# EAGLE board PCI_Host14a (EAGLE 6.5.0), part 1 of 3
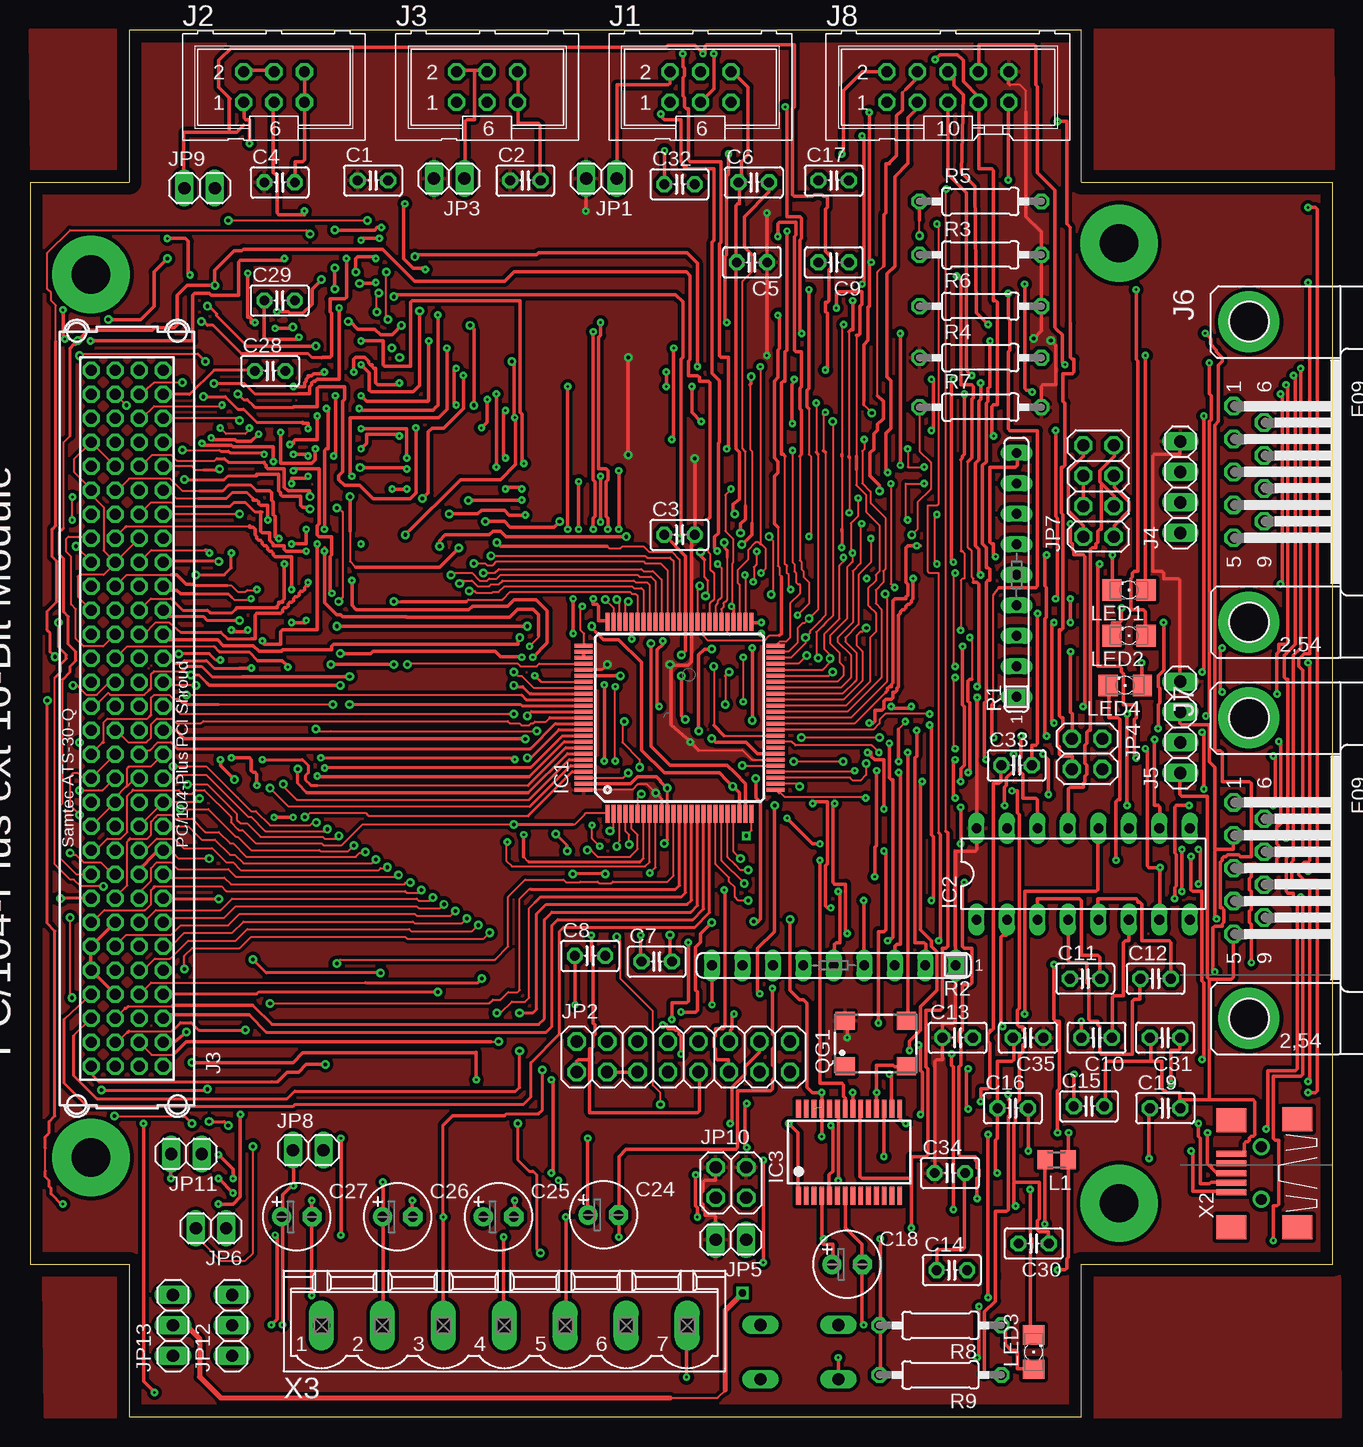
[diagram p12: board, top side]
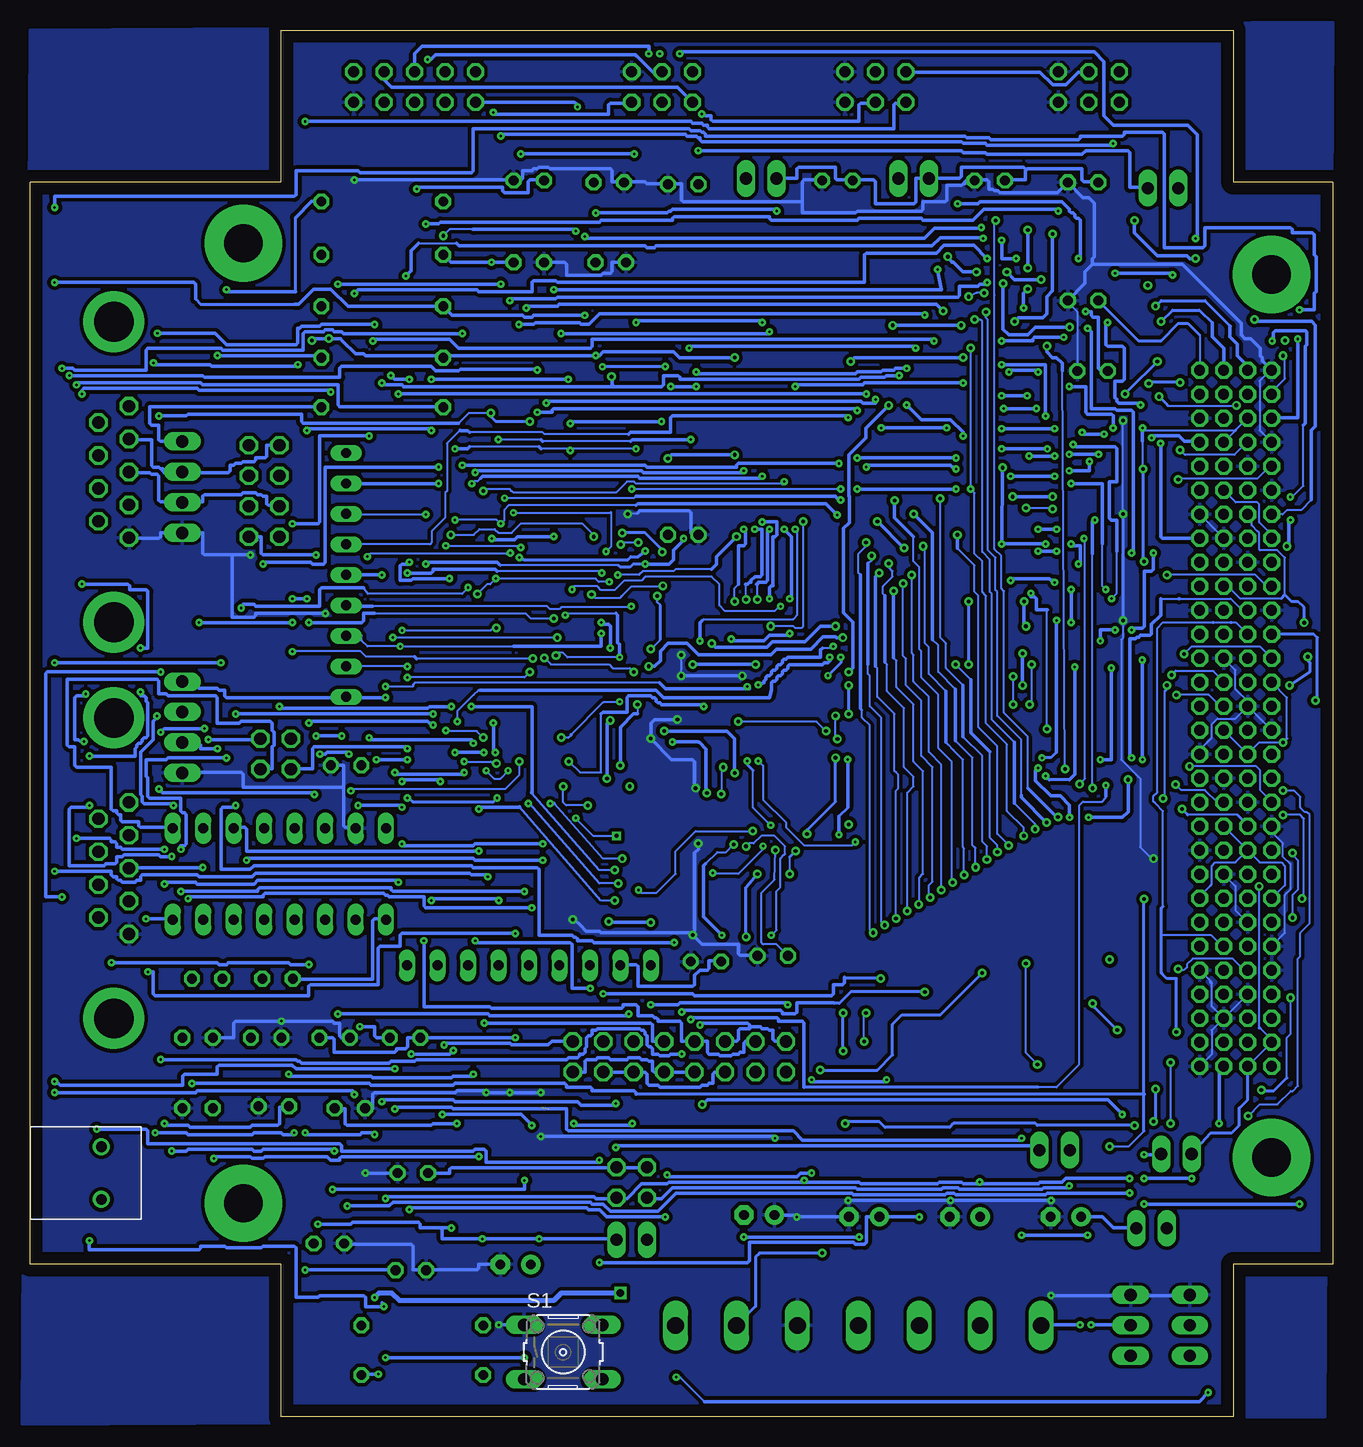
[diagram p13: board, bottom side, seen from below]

Size 108.6 x 115.57 mm. Coordinates in mm from the lower left corner, seen from the top.
Copper layers (1*16): Top 0.035mm / dielectric 1.5mm / Bottom 0.035mm
Design rules "default *": minimum track width 6mil, minimum drill 8mil, track to track 6mil, track to pad 6mil, pad to pad 8mil, via to via 8mil, smd to smd 8mil, copper to edge 40mil, drill to drill 8mil, minimum pad ring 10mil, minimum via ring 8mil, stop-mask expansion 4mil, vias tented up to drill 0mil, thermal gap 10mil
Net classes: 0 default: width 0.152 mm

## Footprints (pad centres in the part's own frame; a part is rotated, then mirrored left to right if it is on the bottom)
C025-025X050 = drill 0.813 octagon: 1 -1.27,0; 2 1.27,0
E2,5-6 = drill 0.813 pad 1.6: + -1.27,0 | drill 0.813 pad 1.6 octagon: - 1.27,0
TQFP100 = smd 1.5 x 0.35: 1 -8,6; 2 -8,5.5; 3 -8,5; 4 -8,4.5; 5 -8,4; 6 -8,3.5; 7 -8,3; 8 -8,2.5; 9 -8,2; 10 -8,1.5; 11 -8,1; 12 -8,0.5; 13 -8,0; 14 -8,-0.5; 15 -8,-1; 16 -8,-1.5; 17 -8,-2; 18 -8,-2.5; 19 -8,-3; 20 -8,-3.5; 21 -8,-4; 22 -8,-4.5; 23 -8,-5; 24 -8,-5.5; 25 -8,-6; 51 8,-6; 52 8,-5.5; 53 8,-5; 54 8,-4.5; 55 8,-4; 56 8,-3.5; 57 8,-3; 58 8,-2.5; 59 8,-2; 60 8,-1.5; 61 8,-1; 62 8,-0.5; 63 8,0; 64 8,0.5; 65 8,1; 66 8,1.5; 67 8,2; 68 8,2.5; 69 8,3; 70 8,3.5; 71 8,4; 72 8,4.5; 73 8,5; 74 8,5.5; 75 8,6 | smd 0.35 x 1.5: 26 -6,-8; 27 -5.5,-8; 28 -5,-8; 29 -4.5,-8; 30 -4,-8; 31 -3.5,-8; 32 -3,-8; 33 -2.5,-8; 34 -2,-8; 35 -1.5,-8; 36 -1,-8; 37 -0.5,-8; 38 0,-8; 39 0.5,-8; 40 1,-8; 41 1.5,-8; 42 2,-8; 43 2.5,-8; 44 3,-8; 45 3.5,-8; 46 4,-8; 47 4.5,-8; 48 5,-8; 49 5.5,-8; 50 6,-8; 76 6,8; 77 5.5,8; 78 5,8; 79 4.5,8; 80 4,8; 81 3.5,8; 82 3,8; 83 2.5,8; 84 2,8; 85 1.5,8; 86 1,8; 87 0.5,8; 88 0,8; 89 -0.5,8; 90 -1,8; 91 -1.5,8; 92 -2,8; 93 -2.5,8; 94 -3,8; 95 -3.5,8; 96 -4,8; 97 -4.5,8; 98 -5,8; 99 -5.5,8; 100 -6,8
DIL16 = drill 0.813 long: 1 -8.89,-3.81; 2 -6.35,-3.81; 3 -3.81,-3.81; 4 -1.27,-3.81; 5 1.27,-3.81; 6 3.81,-3.81; 7 6.35,-3.81; 8 8.89,-3.81; 9 8.89,3.81; 10 6.35,3.81; 11 3.81,3.81; 12 1.27,3.81; 13 -1.27,3.81; 14 -3.81,3.81; 15 -6.35,3.81; 16 -8.89,3.81
SSOP28 = smd 0.4 x 1.5: 1 -4.225,-3.625; 2 -3.575,-3.625; 3 -2.925,-3.625; 4 -2.275,-3.625; 5 -1.625,-3.625; 6 -0.975,-3.625; 7 -0.325,-3.625; 8 0.325,-3.625; 9 0.975,-3.625; 10 1.625,-3.625; 11 2.275,-3.625; 12 2.925,-3.625; 13 3.575,-3.625; 14 4.225,-3.625; 15 4.225,3.625; 16 3.575,3.625; 17 2.925,3.625; 18 2.275,3.625; 19 1.625,3.625; 20 0.975,3.625; 21 0.325,3.625; 22 -0.325,3.625; 23 -0.975,3.625; 24 -1.625,3.625; 25 -2.275,3.625; 26 -2.925,3.625; 27 -3.575,3.625; 28 -4.225,3.625
ML6 = drill 0.914 octagon: 1 -2.54,-1.27; 2 -2.54,1.27; 3 0,-1.27; 4 0,1.27; 5 2.54,-1.27; 6 2.54,1.27
1X04 = drill 1.016 long: 1 -3.81,0; 2 -1.27,0; 3 1.27,0; 4 3.81,0
F09HP = drill 1.016 octagon: 1 -5.486,-1.27; 2 -2.743,-1.27; 3 0,-1.27; 4 2.743,-1.27; 5 5.486,-1.27; 6 -4.115,1.27; 7 -1.372,1.27; 8 1.372,1.27; 9 4.115,1.27 | drill 3.302 pad 5.08: G1 -12.522,0; G2 12.522,0
ML10 = drill 0.914 octagon: 1 -5.08,-1.27; 2 -5.08,1.27; 3 -2.54,-1.27; 4 -2.54,1.27; 5 0,-1.27; 6 0,1.27; 7 2.54,-1.27; 8 2.54,1.27; 9 5.08,-1.27; 10 5.08,1.27
1X02 = drill 1.016 long: 1 -1.27,0; 2 1.27,0
2X08 = drill 1.016 octagon: 1 -8.89,-1.27; 2 -8.89,1.27; 3 -6.35,-1.27; 4 -6.35,1.27; 5 -3.81,-1.27; 6 -3.81,1.27; 7 -1.27,-1.27; 8 -1.27,1.27; 9 1.27,-1.27; 10 1.27,1.27; 11 3.81,-1.27; 12 3.81,1.27; 13 6.35,-1.27; 14 6.35,1.27; 15 8.89,-1.27; 16 8.89,1.27
2X02 = drill 1.016 octagon: 1 -1.27,-1.27; 2 -1.27,1.27; 3 1.27,-1.27; 4 1.27,1.27
2X04 = drill 1.016 octagon: 1 -3.81,-1.27; 2 -3.81,1.27; 3 -1.27,-1.27; 4 -1.27,1.27; 5 1.27,-1.27; 6 1.27,1.27; 7 3.81,-1.27; 8 3.81,1.27
1X03 = drill 1.016 long: 1 -2.54,0; 2 0,0; 3 2.54,0
M0805 = smd 1.3 x 1.6: 1 -0.95,0; 2 0.95,0
1206 = smd 1.6 x 1.803: A -1.422,0; C 1.422,0
SM77H = smd 1.6 x 1.5: 1 -2.55,-1.9; 2 2.55,-1.9; 3 2.55,1.9; 4 -2.55,1.9
SIL9 = drill 0.813 long: 1 -10.16,0; 2 -7.62,0; 3 -5.08,0; 4 -2.54,0; 5 0,0; 6 2.54,0; 7 5.08,0; 8 7.62,0; 9 10.16,0
0207/10 = drill 0.813 octagon: 1 -5.08,0; 2 5.08,0
B3F-10XX = drill 1.016 long: 1 -3.251,2.261; 2 3.251,2.261; 3 -3.251,-2.261; 4 3.251,-2.261
PC104-PLUS = drill 0.9 octagon: J3-A1 11.08,16.51; J3-A2 11.08,18.51; J3-A3 11.08,20.51; J3-A4 11.08,22.51; J3-A5 11.08,24.51; J3-A6 11.08,26.51; J3-A7 11.08,28.51; J3-A8 11.08,30.51; J3-A9 11.08,32.51; J3-A10 11.08,34.51; J3-A11 11.08,36.51; J3-A12 11.08,38.51; J3-A13 11.08,40.51; J3-A14 11.08,42.51; J3-A15 11.08,44.51; J3-A16 11.08,46.51; J3-A17 11.08,48.51; J3-A18 11.08,50.51; J3-A19 11.08,52.51; J3-A20 11.08,54.51; J3-A21 11.08,56.51; J3-A22 11.08,58.51; J3-A23 11.08,60.51; J3-A24 11.08,62.51; J3-A25 11.08,64.51; J3-A26 11.08,66.51; J3-A27 11.08,68.51; J3-A28 11.08,70.51; J3-A29 11.08,72.51; J3-A30 11.08,74.51; J3-B1 9.08,16.51; J3-B2 9.08,18.51; J3-B3 9.08,20.51; J3-B4 9.08,22.51; J3-B5 9.08,24.51; J3-B6 9.08,26.51; J3-B7 9.08,28.51; J3-B8 9.08,30.51; J3-B9 9.08,32.51; J3-B10 9.08,34.51; J3-B11 9.08,36.51; J3-B12 9.08,38.51; J3-B13 9.08,40.51; J3-B14 9.08,42.51; J3-B15 9.08,44.51; J3-B16 9.08,46.51; J3-B17 9.08,48.51; J3-B18 9.08,50.51; J3-B19 9.08,52.51; J3-B20 9.08,54.51; J3-B21 9.08,56.51; J3-B22 9.08,58.51; J3-B23 9.08,60.51; J3-B24 9.08,62.51; J3-B25 9.08,64.51; J3-B26 9.08,66.51; J3-B27 9.08,68.51; J3-B28 9.08,70.51; J3-B29 9.08,72.51; J3-B30 9.08,74.51; J3-C1 7.08,16.51; J3-C2 7.08,18.51; J3-C3 7.08,20.51; J3-C4 7.08,22.51; J3-C5 7.08,24.51; J3-C6 7.08,26.51; J3-C7 7.08,28.51; J3-C8 7.08,30.51; J3-C9 7.08,32.51; J3-C10 7.08,34.51; J3-C11 7.08,36.51; J3-C12 7.08,38.51; J3-C13 7.08,40.51; J3-C14 7.08,42.51; J3-C15 7.08,44.51; J3-C16 7.08,46.51; J3-C17 7.08,48.51; J3-C18 7.08,50.51; J3-C19 7.08,52.51; J3-C20 7.08,54.51; J3-C21 7.08,56.51; J3-C22 7.08,58.51; J3-C23 7.08,60.51; J3-C24 7.08,62.51; J3-C25 7.08,64.51; J3-C26 7.08,66.51; J3-C27 7.08,68.51; J3-C28 7.08,70.51; J3-C29 7.08,72.51; J3-C30 7.08,74.51; J3-D1 5.08,16.51; J3-D2 5.08,18.51; J3-D3 5.08,20.51; J3-D4 5.08,22.51; J3-D5 5.08,24.51; J3-D6 5.08,26.51; J3-D7 5.08,28.51; J3-D8 5.08,30.51; J3-D9 5.08,32.51; J3-D10 5.08,34.51; J3-D11 5.08,36.51; J3-D12 5.08,38.51; J3-D13 5.08,40.51; J3-D14 5.08,42.51; J3-D15 5.08,44.51; J3-D16 5.08,46.51; J3-D17 5.08,48.51; J3-D18 5.08,50.51; J3-D19 5.08,52.51; J3-D20 5.08,54.51; J3-D21 5.08,56.51; J3-D22 5.08,58.51; J3-D23 5.08,60.51; J3-D24 5.08,62.51; J3-D25 5.08,64.51; J3-D26 5.08,66.51; J3-D27 5.08,68.51; J3-D28 5.08,70.51; J3-D29 5.08,72.51; J3-D30 5.08,74.51 | drill 3.2 pad 6.452: P$1 5.085,82.5; P$2 5.085,8.9; P$3 90.785,5.1; P$4 90.785,85.1
USB-MB-S = smd 2.5 x 0.5: D+ 2.5,0; D- 2.5,0.8; GND 2.5,-1.6; ID 2.5,-0.8; VBUS 2.5,1.6 | smd 2.5 x 2: P$1 -3,-4.5; P$2 -3,4.5; P$3 2.5,-4.4; P$4 2.5,4.5 | drill 0.9: P$5 0,2.2; P$6 0,-2.2
MSTBV7 = drill 1.397 long: 1 -15.24,0; 2 -10.16,0; 3 -5.08,0; 4 0,0; 5 5.08,0; 6 10.16,0; 7 15.24,0

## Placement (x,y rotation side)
C1  100nF  [C025-025X050]  28.59,103.03 0 top
C2  100nF  [C025-025X050]  41.29,103.03 0 top
C3  100nF  [C025-025X050]  54.15,73.5 0 top
C4  100nF  [C025-025X050]  20.81,102.87 0 top
C5  100nF  [C025-025X050]  60.18,96.2 180 top
C6  100nF  [C025-025X050]  60.34,102.87 0 top
C7  10n  [C025-025X050]  52.24,37.94 0 top
C8  10n  [C025-025X050]  46.69,38.42 0 top
C9  10n  [C025-025X050]  67.01,96.2 180 top
C10  1u  [C025-025X050]  88.92,31.59 180 top
C11  1u  [C025-025X050]  87.96,36.51 0 top
C12  1u  [C025-025X050]  93.84,36.51 0 top
C13  1u  [C025-025X050]  77.33,31.59 0 top
C14  10n  [C025-025X050]  76.85,12.22 0 top
C15  47p  [C025-025X050]  88.28,25.88 0 top
C16  47p  [C025-025X050]  81.93,25.72 0 top
C17  100n  [C025-025X050]  67.01,103.03 0 top
C18  4.7u  [E2,5-6]  68.12,12.7 0 top
C19  100n  [C025-025X050]  94.63,25.72 0 top
C24  47u  [E2,5-6]  47.8,16.83 0 top
C25  47u  [E2,5-6]  39.07,16.67 0 top
C26  47u  [E2,5-6]  30.65,16.67 0 top
C27  47u  [E2,5-6]  22.24,16.67 0 top
C28  100n  [C025-025X050]  20.02,87.15 0 top
C29  100n  [C025-025X050]  20.81,93.03 0 top
C30  100n  [C025-025X050]  83.68,14.45 180 top
C31  100n  [C025-025X050]  94.63,31.59 180 top
C32  100n  [C025-025X050]  54.15,102.71 0 top
C33  100n  [C025-025X050]  82.25,54.29 0 top
C34  100n  [C025-025X050]  76.69,20.32 0 top
C35  100n  [C025-025X050]  83.2,31.59 180 top
IC1  ATMEGA640-16AI  [TQFP100]  54.15,58.26 90 top
IC2  MAX232  [DIL16]  87.8,45.24 0 top
IC3  FT232RL  [SSOP28]  68.28,22.07 0 top
J1  [ML6]  55.9,110.81 0 top
J2  [ML6]  20.34,110.81 0 top
J3  [ML6]  38.12,110.81 0 top
J4  [1X04]  95.9,77.47 90 top
J5  [1X04]  95.9,57.47 90 top
J6  [F09HP]  101.61,78.74 270 top
J7  [F09HP]  101.61,45.72 270 top
J8  [ML10]  76.53,110.81 0 top
JP1  [1X02]  47.64,103.19 180 top
JP2  [2X08]  54.47,30 0 top
JP3  [1X02]  34.94,103.19 180 top
JP4  [2X02]  88.12,55.24 270 top
JP5  [1X02]  58.44,14.76 180 top
JP6  [1X02]  15.1,15.72 180 top
JP7  [2X04]  89.07,77.15 90 top
JP8  [1X02]  23.19,22.23 0 top
JP9  [1X02]  14.14,102.39 0 top
JP10  [2X02]  58.43,19.53 0 top
JP11  [1X02]  13.03,21.91 180 top
JP12  [1X03]  16.84,7.62 90 top
JP13  [1X03]  11.92,7.62 90 top
L1  [M0805]  85.58,21.43 180 top
LED1  gr  [1206]  91.61,68.9 180 top
LED2  [1206]  91.61,65.09 180 top
LED3  rt  [1206]  83.68,5.4 90 top
LED4  or  [1206]  91.3,60.96 180 top
QG1  SM77H  [SM77H]  70.5,31.11 0 top
R1  4K7  [SIL9]  82.25,70.17 90 top
R2  4k7  [SIL9]  67.01,37.62 180 top
R3  10k  [0207/10]  79.23,96.84 0 top
R4  220R  [0207/10]  79.23,88.27 0 top
R5  220R  [0207/10]  79.23,101.28 0 top
R6  10k  [0207/10]  79.23,92.55 0 top
R7  10k  [0207/10]  79.23,84.14 0 top
R8  220R  [0207/10]  75.9,7.62 180 top
R9  220R  [0207/10]  75.9,3.49 180 top
S1  [B3F-10XX]  64.15,5.4 0 bottom
X1  PC104_PLUS_USB_SUBD  [PC104-PLUS]  0.01,12.7 0 top
X2  USB-MB-S  [USB-MB-S]  102.65,20.32 180 top
X3  MSTBV7  [MSTBV7]  39.54,7.62 0 top

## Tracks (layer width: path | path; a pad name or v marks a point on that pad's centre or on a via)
AD00  (via drill 0.3)
  Top 0.152: v25.57,37.78 25.89,38.1 38.75,38.1 39.86,39.21 39.86,43.34 41.29,44.77 44.47,44.77 44.7,44.53 45.81,44.53 45.89,44.61 47.32,44.61 47.48,44.45 48.43,44.45 48.59,44.61 53.15,44.61 53.65,45.11 IC1.12
  Top 0.254: X1.J3-D1 5.09,28.57 5.73,27.94 20.18,27.94 20.65,27.94
  Top 0.305: v24.62,29.37 23.03,29.37 22.4,28.73 21.45,28.73 20.65,27.94
  Bottom 0.152: v24.62,29.37 25.57,30.32 v25.57,37.78
AD01  (via drill 0.3)
  Top 0.152: 7.25,31.21 8.11,32.07 | 8.27,32.15 11.84,32.15 | v20.02,34.45 38.27,34.45 38.59,34.77 39.23,34.77 39.86,35.4 40.66,35.4 40.81,35.56 40.81,43.18 41.61,43.97 41.77,43.97
  Top 0.254: X1.J3-C2 7.25,31.21 | 8.11,32.07 8.19,32.07 8.27,32.15 | 11.84,32.15 12.56,32.86 13.43,32.86 14.06,32.23 v17.95,32.23 | IC1.13 54.15,44.29 53.83,43.97 41.77,43.97
  Top 0.305: v20.02,34.45 | v20.02,34.45 19.98,34.49
  Bottom 0.254: v17.95,32.23 19.86,34.13
  Bottom 0.305: 19.86,34.13 20.02,34.29 v20.02,34.45
AD02  (via drill 0.3)
  Top 0.152: 11.92,30.16 10.14,30.16 X1.J3-B2 | 42.08,42.86 41.61,42.39 41.61,34.92 41.29,34.61 40.18,34.61 39.23,33.66 v38.91,33.66 | 38.43,31.27 v39.07,31.27
  Top 0.254: IC1.14 54.65,43.68 54.31,43.34 42.56,43.34 42.08,42.86
  Top 0.305: 38.43,31.27 13.03,31.27 11.92,30.16
  Bottom 0.152: v38.91,33.66 39.07,33.5 v39.07,31.27
AD03  (via drill 0.3)
  Top 0.152: 3.67,31.78 X1.J3-D3
  Top 0.254: IC1.15 55.15,43.07 54.78,42.7 43.04,42.7 | 3.67,31.78 3.67,28.42 5.57,26.51 21.45,26.51 22.08,27.15 40.5,27.15 40.81,27.46 v40.81,30.48 | v40.81,33.66 41.92,33.66 42.24,33.97 42.24,41.91 43.04,42.7 | 43.04,42.7
  Bottom 0.254: v40.81,30.48 v40.81,33.66
AD04
  Top 0.152: 8.19,34.21 11.84,34.21 | X1.J3-C3 7.94,34.05
  Top 0.254: IC1.16 55.65,42.62 55.1,42.07 43.51,42.07 42.88,41.43 42.88,33.18 42.4,32.7 20.17,32.7 18.58,34.29 | 8.19,34.21 8.03,34.05 7.94,34.05
  Top 0.305: 18.58,34.29 11.92,34.29 11.84,34.21
AD05
  Top 0.254: IC1.17 56.15,42.32 55.26,41.43 43.99,41.43 43.51,40.96 43.51,32.54 43.04,32.07 19.7,32.07 18.27,33.5
  Top 0.305: 18.27,33.5 11.38,33.5 X1.J3-A3
AD06
  Top 0.152: 2.87,33.15 X1.J3-D4
  Top 0.254: IC1.18 56.65,42.03 55.42,40.8 44.47,40.8 44.15,40.48 44.15,31.91 41.77,29.53 41.77,26.67 41.13,26.04 22.08,26.04 21.92,25.88 4.78,25.88 2.87,27.78 2.87,33.15
AD07  (via drill 0.2, 0.3)
  Top 0.152: 9.11,35.21 10.1,36.2 27.96,36.2 | IC1.27 63.91,52.76 v64.15,52.53
  Top 0.254: X1.J3-B4 9.11,35.21 | 27.96,36.2 37.34,36.2 v37.68,36.54
  Top 0.305: v62.09,50.96 62.04,50.95 62.04,40.44 60.66,39.05 60.66,35.42 v60.82,35.25
  Bottom 0.152: v64.15,52.53 64.15,51.2 63.91,50.96 v62.09,50.96
  Bottom 0.254: v37.68,36.54 40.62,36.54 40.71,36.63
  Bottom 0.305: v60.82,35.25 53.36,35.25 53.2,35.1 41.77,35.1 41.62,35.25 41.62,36.02 40.86,36.02 40.71,36.17 40.71,36.63
AD08  (via drill 0.3)
  Top 0.152: 51.13,72.55 51.61,72.07 53.51,72.07 54.15,71.44 IC1.63 | IC1.63 | 51.13,72.55 | v12.87,37.31 12.87,38.42 13.51,39.05 17.48,39.05 18.43,40 31.29,40 31.45,39.85 37.82,39.85 v38.31,40.34 | 48.12,72.55 48.27,72.39 | 48.27,72.39 | 48.27,72.39 49.23,72.39 49.39,72.55 51.13,72.55
  Top 0.305: v38.91,72.87 39.23,72.55 48.12,72.55
  Bottom 0.152: 7.38,37.21 8.35,38.18 11.68,38.18 12.16,37.7 12.16,37.47 12.4,37.23 12.64,37.23 | v38.31,40.34 38.59,40.62 38.59,57.63 39.23,58.26 39.23,58.9 39.38,59.05 | 39.38,70.17 39.54,70.33 39.54,71.91 38.91,72.55 v38.91,72.87
  Bottom 0.254: X1.J3-C5 7.38,37.21 | 12.64,37.23 12.71,37.31 v12.87,37.31
  Bottom 0.305: 39.38,59.05 39.38,70.17
AD09  (via drill 0.3)
  Top 0.152: X1.J3-B5 9.44,37.21 10.41,38.18 11.68,38.18 13.19,39.69 17.16,39.69 18.11,40.64 31.61,40.64 31.77,40.48 36.87,40.48 v37.36,40.97 | v38.43,71.75 51.29,71.75 51.45,71.6 53.36,71.6 53.67,71.28 53.65,71.25 IC1.64
  Bottom 0.152: v37.36,40.97 37.64,41.25 37.64,58.26 38.59,59.21 38.59,61.75 38.75,61.91 38.75,62.55 38.75,62.71 | 38.75,71.12 38.43,71.44 v38.43,71.75
  Bottom 0.305: 38.75,62.71 38.75,71.12
AD10  (via drill 0.3)
  Top 0.152: 7.09,39.23 8.03,40.16 11.76,40.16 12.08,40.48 | v37,71.12 37.32,71.12 | 37.32,71.12 | 37.32,71.12 37.96,71.12 38.12,70.96 38.59,70.96 38.91,71.28 51.13,71.28 51.29,71.12 52.56,71.12 53.15,70.53 IC1.65 | 12.08,40.48 | 12.08,40.48 12.56,40.96 16.53,40.96 17.48,41.91 32.08,41.91 32.24,41.75 35.06,41.75 v35.46,42.15
  Top 0.254: X1.J3-C6 7.09,39.23
  Bottom 0.152: 37.32,68.42 37.48,68.58 37.48,69.22 36.69,70.01 36.69,70.48 37,70.8 v37,71.12 | 37.32,62.86 37.16,62.71 37.16,60.48 35.73,59.05 35.73,54.13 34.94,53.34 34.94,52.55 35.46,52.02 v35.46,42.15
  Bottom 0.305: 37.32,62.86 37.32,68.42
AD11  (via drill 0.3)
  Top 0.152: 52.24,70.17 | v37.8,70.33 38.75,70.33 39.07,70.64 50.97,70.64 51.13,70.48 51.93,70.48 52.24,70.17 | X1.J3-A6 11.76,39.21 12.87,40.32 16.84,40.32 17.8,41.27 31.92,41.27 32.08,41.12 36.01,41.12 v36.41,41.52 | IC1.66 52.65,69.76 52.24,70.17
  Bottom 0.152: v37.8,70.33 | 38.12,70.01 v37.8,70.33 | 38.12,62.55 37.96,62.39 37.96,60.01 36.53,58.58 36.53,53.82 36.37,53.66 | 36.37,53.66 | 36.37,53.66 36.21,53.5 36.21,52.39 36.41,52.19 v36.41,41.52
  Bottom 0.305: 38.12,62.55 38.12,70.01
AD12  (via drill 0.3)
  Top 0.152: 5.19,41.21 6.21,42.23 9.54,42.23 9.62,42.23 10.1,42.7 10.1,43.89 10.33,44.13 | 10.41,44.21 15.97,44.21 16.37,43.81 31.29,43.81 31.45,43.66 32.37,43.66 v32.62,43.91 | v35.1,70.17 35.26,70.33 36.84,70.33 37.48,69.69 38.12,69.69 38.27,69.85 38.91,69.85 39.23,70.17 50.66,70.17 50.81,70.01 51.77,70.01 52.15,69.63 IC1.67
  Top 0.254: X1.J3-D7 5.19,41.21 | 10.33,44.13 | 10.33,44.13 10.41,44.21
  Bottom 0.152: v32.62,43.91 32.62,54.36 33.67,55.4 33.67,60.01 34.94,61.28 34.94,63.5 35.1,63.66 v35.1,70.17
AD13  (via drill 0.3)
  Top 0.152: X1.J3-B7 9.48,41.21 10.49,42.23 15.89,42.23 16.84,43.18 32.24,43.18 32.4,43.02 33.33,43.02 v33.57,43.27 | v35.81,69.45 36.05,69.69 36.84,69.69 37.32,69.22 38.27,69.22 38.43,69.37 39.07,69.37 39.38,69.69 50.34,69.69 50.5,69.53 51.45,69.53 51.65,69.33 IC1.68
  Bottom 0.152: v35.81,69.45 35.81,63.42 35.58,63.18 35.58,60.96 34.3,59.69 34.3,55.09 33.35,54.13 33.35,44.61 33.67,44.29 33.67,43.36 v33.57,43.27
AD14  (via drill 0.3)
  Top 0.152: 38.59,68.74 39.07,68.74 39.54,69.22 50.18,69.22 50.34,69.06 50.97,69.06 51.15,68.88 IC1.69 | 38.59,68.74 | 38.59,68.74 38.51,68.66 37.24,68.66 37.08,68.82 v36.61,68.82 | X1.J3-A7 11.54,41.21 11.92,41.59 16.21,41.59 17.16,42.55 32.24,42.55 32.4,42.39 34.19,42.39 v34.52,42.71
  Bottom 0.152: v34.52,42.71 34.46,42.76 34.46,44.93 34.15,45.24 34.15,53.82 34.94,54.61 34.94,59.37 36.37,60.8 36.37,63.02 36.61,63.26
  Bottom 0.305: 36.61,63.26 v36.61,68.82
AD15  (via drill 0.3)
  Top 0.152: 7.09,43.35 8.11,44.29 8.11,47.94 8.27,48.1 | 8.35,48.18 9.78,48.18 10.1,48.5 10.1,49.61 10.49,50.01 10.65,50.17 11.76,50.17 12.08,49.85 13.51,49.85 14.62,48.74 15.73,48.74 16.68,47.78 16.92,47.78 18.03,46.67 27.16,46.67 27.48,46.99 27.88,46.99 v27.96,47.07 | IC1.79 42.46,62.76 42.24,62.55 40.89,62.55 40.66,62.79 31.53,62.79 v31.45,62.71
  Top 0.254: X1.J3-C8 7.09,43.35 | 8.27,48.1 | 8.27,48.1 8.35,48.18
  Bottom 0.152: v27.96,47.07 27.96,47.62 28.59,48.26 28.59,55.4 | 30.18,61.44 v31.45,62.71
  Bottom 0.305: 28.59,55.4 30.18,56.99 30.18,61.44
AD16
  Top 0.152: 9.45,55.56 10.02,55.56 10.65,56.2 11.76,56.2
  Top 0.254: X1.J3-B14 9.45,55.56 | 11.76,56.2 12.28,55.68 41.72,55.68 43.82,57.78 43.85,57.76 IC1.89
AD17
  Top 0.152: 7.18,57.21 8.19,56.2 9.7,56.2 10.1,56.59 10.1,57.71 10.57,58.18 11.84,58.18 12.24,57.78 14.24,57.78 14.44,57.98 39.82,57.98 40.02,57.78 40.81,57.78 40.97,57.63 41.61,57.63 41.77,57.78 41.92,57.78 42.08,57.94 43.04,57.94 43.35,58.26
  Top 0.254: X1.J3-C15 7.18,57.21 | IC1.88 43.35,58.26
AD18  (via drill 0.3)
  Top 0.254: X1.J3-A15 12.18,57.21 | 41.77,58.74 v41.45,58.42 41.79,58.76 IC1.87
  Top 0.305: 12.18,57.21 12.87,56.52 41.27,56.52 v41.29,56.5
  Bottom 0.152: v41.45,58.42 41.45,56.65 v41.29,56.5
AD19  (via drill 0.3)
  Top 0.152: X1.J3-D16 5.41,59.21 6.52,60.33 6.68,60.17 9.54,60.17 9.94,60.56 | 10.1,60.72 10.1,61.91 10.33,62.15 12.71,62.15 | v26.64,61.69 26.39,61.69 26.37,61.67
  Top 0.254: 9.94,60.56 | 9.94,60.56 10.1,60.72 | 12.71,62.15 13.11,62.55 14.3,62.55 15.18,61.67 17.72,61.67 | v26.64,59.37 40.89,59.37 41,59.26 IC1.86 | 26.45,61.67
  Top 0.305: 17.72,61.67 26.37,61.67 26.45,61.67
  Bottom 0.152: v26.64,61.69 v26.64,59.37
AD20  (via drill 0.3)
  Top 0.152: v13.03,60.17 40.97,60.17
  Top 0.254: 40.97,60.17 41.37,59.77 IC1.85
  Bottom 0.152: 9.38,59.21 10.33,60.17 v13.03,60.17
  Bottom 0.254: X1.J3-B16 9.38,59.21
AD21  (via drill 0.3)
  Top 0.152: v40.34,58.58 12.52,58.58 11.89,59.21 X1.J3-A16
  Top 0.254: 41.79,60.26 IC1.84 | 41.79,60.26 41.79,60.27 | 41.33,60.58 | 41.33,60.58 41.07,60.84 40.46,60.84 v40.34,60.96 | 41.79,60.26 41.65,60.26 41.33,60.58
  Bottom 0.254: v40.34,58.58 v40.34,60.96
AD22  (via drill 0.3)
  Top 0.152: X1.J3-C17 6.61,61.21 5.57,60.17 4.7,60.17 3.9,60.96 | IC1.83 41.97,60.76 40.97,61.75 40.66,61.75 v40.34,62.07 | 2.16,89.61 2.16,92.63 1.76,93.03 1.76,93.66 1.44,93.98 1.44,97 3.35,98.9 23.03,98.9 v23.35,98.58
  Top 0.254: 2.16,89.61 2.16,74.3 1.84,73.98 1.84,71.68 2.24,71.28 2.24,67.94 1.44,67.15 1.44,65.56 1.68,65.33 1.68,63.74 v2.08,63.34 | v3.59,60.96 3.9,60.96
  Top 0.305: v37,84.3 37,90.65 v36.69,90.96 | v26.53,91.28 26.69,91.28 27.32,90.65 28.75,90.65 29.23,90.17 30.18,90.17 v30.97,90.96
  Bottom 0.254: v3.59,60.96 1.92,62.07 1.92,62.86 2.08,63.02 v2.08,63.34
  Bottom 0.305: v37,84.3 38.91,82.39 38.91,81.6 40.34,80.17 40.34,76.74 40.3,76.7 40.3,74.51 40.77,74.04 40.77,67.01 39.98,66.22 39.98,62.43 v40.34,62.07 | v30.97,90.96 v36.69,90.96 | v23.35,98.58 23.35,93.82 23.83,93.34 23.83,91.92 24.14,91.6 26.21,91.6 v26.53,91.28
AD23  (via drill 0.2, 0.3)
  Top 0.152: 42.59,61.26 IC1.82
  Top 0.254: v13.43,61.83 14.07,61.83 14.78,61.12 | v42.08,61.76 42.08,61.77 42.59,61.26
  Top 0.305: v25.86,60.96 25.54,60.96 14.94,60.96 14.78,61.12 | v25.86,63.61 28.38,63.61 28.59,63.82 38.75,63.82 39.23,63.34 40.97,63.34 v41.01,63.3
  Bottom 0.152: 9.1,61.31 9.94,62.15 13.11,62.15
  Bottom 0.254: X1.J3-B17 9.1,61.31 | 13.11,62.15 v13.43,61.83 | v41.01,63.3 41.01,62.83 v42.08,61.76
  Bottom 0.305: v25.86,60.96 v25.86,63.61
AD24  (via drill 0.3)
  Top 0.152: v57.01,62.55 57.01,57.63 | 57.87,56.76 IC1.35
  Top 0.305: X1.J3-A19 11.16,65.21 11.6,64.77 15.65,64.77 16.12,64.27 18.61,64.27 19.09,63.82 20.97,63.82 21.05,63.91 25.16,63.91 25.16,64.21 25.31,64.36 40.71,64.36 40.71,64.82 v40.83,64.93 | 57.01,57.63 57.87,56.76
  Bottom 0.305: v57.01,62.55 56.53,62.55 56.05,63.02 56.05,63.82 55.42,64.45 53.83,64.45 52.88,63.5 46.85,63.5 46.37,63.98 43.51,63.98 42.48,65.01 41.45,65.01 41.37,64.93 v40.83,64.93
AD25  (via drill 0.2)
  Top 0.152: IC1.36 70.29,57.26 70.82,57.78 70.82,58.1 71.29,58.58 v74.99,58.58 v75,58.57
  Top 0.305: v91.45,50.95 v91.45,58.57 | v54.88,39.52 54.88,34.65 54.73,34.49 53.51,34.49 v53.51,33.12 | v18.91,52.63 18.91,53.54 18.76,53.7 18.61,53.7 18.46,53.85 18.46,54.76 18.3,54.92 v16.78,54.92
  Bottom 0.152: 7.63,67.31 8.51,68.18 12.79,68.18 | 18.91,51.71 18.91,51.59 19.22,51.28 20.81,51.28 21.13,50.96 21.13,29.37 23.03,27.46 24.53,27.46 24.55,27.48 | 14.34,68.17 12.82,68.17
  Bottom 0.254: 7.63,67.31 7.19,67.31 X1.J3-C20 | 24.55,27.48 44.06,27.48
  Bottom 0.305: v91.45,58.57 v75,58.57 | v91.45,50.95 91.61,50.8 92.52,50.8 92.67,50.65 92.67,45.62 90.24,45.62 89.93,45.92 71.8,45.92 71.64,45.77 66.31,45.77 66.16,45.62 66.16,40.13 63.41,40.13 63.26,39.98 63.11,39.98 62.96,39.83 62.96,39.67 61.74,39.67 61.59,39.52 v54.88,39.52 | v53.51,33.12 53.36,33.27 46.34,33.27 46.19,33.12 46.19,32.97 44.21,32.97 44.06,32.82 44.06,27.48 | 18.91,51.71 v18.91,52.63 | 14.34,68.17 14.34,66.8 15.1,66.04 15.1,65.28 15.26,65.13 16.02,65.13 16.17,64.97 16.32,64.97 16.47,64.82 16.93,64.82 16.93,55.07 v16.78,54.92 | 12.82,68.17 12.79,68.18
AD26  (via drill 0.2)
  Top 0.152: X1.J3-B20 10.07,68.18 11.76,68.18 | 67.68,90.88 67.68,80.21 | 67.69,80.06 67.69,73.97 | IC1.37 68.73,57.76 71.29,60.33 | 71.29,60.33 | 71.29,60.33 71.35,60.39 71.45,60.48
  Top 0.254: 11.76,68.18 12.71,67.23 14.78,67.23 15.02,66.99 16.84,66.99 17.16,67.31 | 67.68,73.81 67.68,72.6 v67.67,72.43
  Top 0.305: v24.7,84.02 24.86,83.87 24.86,80.67 24.7,80.67 24.55,80.52 v24.55,73.97 | v67.83,91.03 67.68,90.88 | 67.68,80.21 67.69,80.06 | 67.69,73.97 67.68,73.81 | 74.23,72.59 v73.93,72.59 73.17,72.59 73.02,72.44 73.02,69.55 73.17,69.39 73.17,68.48 73.02,68.33 73.02,68.17 72.1,68.17 71.95,68.02 71.95,61.16 71.8,61.01 71.8,60.86 71.64,60.86 71.49,60.71 71.49,60.55 71.34,60.4 71.35,60.39 | v34,91.82 34,84.31 33.83,84.14 | 33.83,84.14 | 33.83,84.14 33.59,83.9 27.56,83.9 v27.44,84.02 | v21.2,71.07 21.2,68.17 21.05,68.02 21.05,67.87 20.74,67.87 20.74,67.72 20.59,67.56 20.59,67.41 17.24,67.41 17.16,67.31 | v21.81,72.75 23.03,72.75 v23.03,73.97
  Bottom 0.152: 67.96,72.55 73.89,72.55 v73.93,72.59
  Bottom 0.254: v67.67,72.43 67.85,72.43 67.96,72.55
  Bottom 0.305: v24.7,84.02 v27.44,84.02 | v67.83,91.03 66.61,91.03 66.46,91.19 62.8,91.19 62.65,91.03 62.02,91.03 61.13,91.92 34.1,91.92 v34,91.82 | v21.2,71.07 21.05,71.22 21.05,72.59 21.66,72.59 v21.81,72.75 | v23.03,73.97 v24.55,73.97
AD27  (via drill 0.2, 0.3)
  Top 0.152: IC1.38 | 68.3,79.91 v68.3,75.34 v68.29,75.34 | 68.29,90.42 68.29,80.06 | IC1.38 68.44,58.26 71.45,61.28 71.45,68.42 v71.29,68.58 | v60.58,72.1 60.58,71.04 60.34,70.8 60.34,69.62 v60.3,69.58
  Top 0.254: v13.83,70.17 16.21,70.17 16.78,70.74 v16.78,71.98
  Top 0.305: 68.29,80.06 68.3,79.91 | 68.29,90.42 68.44,90.58 68.59,90.58 v68.59,93.02 | v20.43,90.71 21.83,90.71 v21.92,90.81 | v27.48,94.46 28.74,94.46 v28.82,94.54
  Bottom 0.152: X1.J3-D21 5.49,69.21 6.44,70.17 v13.83,70.17 | 68.3,75.56 68.29,75.56 v68.29,75.34 v68.28,75.34 60.24,75.34 60.17,75.41 60.17,72.51 v60.58,72.1 | v60.3,69.58 61.19,69.58 61.29,69.69 | 61.29,69.69 | 61.29,69.69 61.45,69.85 v69.76,69.85 70.23,69.37 70.5,69.37 v71.29,68.58
  Bottom 0.305: v68.59,93.02 68.44,93.17 64.78,93.17 64.63,93.32 31.26,93.32 31.11,93.47 31.11,94.23 29.58,94.23 29.43,94.39 28.97,94.39 v28.82,94.54 | v16.78,71.98 16.63,71.98 16.63,83.72 16.78,83.87 18,83.87 18.15,84.02 20.13,84.02 20.13,90.41 v20.43,90.71 | v21.92,90.81 24.78,90.81 25.41,90.17 27,90.17 27.48,90.65 v27.48,94.46
AD28  (via drill 0.2)
  Top 0.152: X1.J3-C21 8.05,70.17 11.76,70.17 | IC1.39 68.14,58.76 68.75,59.37 70.98,61.59 70.98,67.31 70.5,67.79 70.5,68.9 71.14,69.53 71.14,70.48 71.29,70.64 71.29,74.93 70.08,76.14 | v69.55,81.43 69.55,80.64 69.39,80.49 69.39,77.79 70.08,77.09 70.08,76.14 | 16.45,69.29 16.76,69.29 17.32,68.74 17.95,68.74 18.11,68.9 18.88,68.9 v18.92,68.94 | 70.08,76.14
  Top 0.254: 13.67,69.29 16.45,69.29
  Top 0.305: v53.51,81.43 53.66,81.59 v53.66,89.05 | v26.84,78.38 26.69,78.54 26.69,83.26 34.06,83.26 34.78,83.98 | v23.18,78.38 23.03,78.23 21.81,78.23 v21.81,77.78 | 34.78,83.98 34.78,89.03 v34.76,89.05 | 34.78,83.98 | 11.76,70.17 12.24,70.17 13.03,69.37 13.59,69.37 13.67,69.29
  Bottom 0.152: 66,81.43 v69.55,81.43 | 58.54,81.28 65.85,81.28 | 19.22,72.75 19.22,69.23 v18.92,68.94
  Bottom 0.305: 65.85,81.28 66,81.43 | 58.54,81.28 58.38,81.43 v53.51,81.43 | v53.66,89.05 53.51,89.2 34.91,89.2 v34.76,89.05 | v23.18,78.38 v26.84,78.38 | 19.22,72.75 19.22,77.78 v21.81,77.78
AD29  (via drill 0.2, 0.3)
  Top 0.152: 68.9,90.12 68.9,80.06 | IC1.40 68.01,59.26 70.02,61.28 70.02,64.93 70.5,65.41 70.5,66.99 70.02,67.47 | 68.89,78.96 68.89,77.65 69.71,76.84 69.71,75.41 70.34,74.77 | 70.02,67.47 69.86,67.63 69.86,69.06 70.5,69.69 70.5,70.17 70.82,70.48 70.82,74.3 70.34,74.77 | 70.02,67.47 | 16.78,68.33 | 16.78,68.33 17,68.1 18.35,68.1 v18.43,68.18 | 70.34,74.77
  Top 0.254: X1.J3-A21 11.41,68.9 | 13.51,68.58 16.53,68.58 16.78,68.33
  Top 0.305: v23.94,83.41 23.94,81.43 22.11,81.43 21.96,81.28 21.96,81.13 21.66,81.13 v21.65,81.03 | v67.22,92.41 67.22,93.62 67.38,93.78 69.36,93.78 69.36,92.71 69.2,92.56 69.2,90.27 69.05,90.12 68.9,90.12 | 68.9,80.06 68.89,78.96 | v27.6,87.68 28.27,87.01 28.27,85.57 28.43,85.41 31.92,85.41 32.48,85.96 v32.48,92.15 | 11.41,68.9 12.24,68.9 12.56,68.58 13.51,68.58
  Bottom 0.152: 18,72.14 18,68.61 v18.43,68.18
  Bottom 0.305: 18,72.14 18,74.73 18.46,74.73 18.61,74.88 18.61,77.93 18,77.93 18,80.67 18.15,80.82 21.35,80.82 21.5,80.98 v21.65,81.03 | v23.94,83.41 23.94,87.68 v27.6,87.68 | v67.22,92.41 67.07,92.56 64.63,92.56 64.48,92.71 33.04,92.71 v32.48,92.15
AD30  (via drill 0.2, 0.3)
  Top 0.152: X1.J3-B22 10.12,72.23 14.62,72.23 | 77.59,79.76 77.59,72.14 77.74,72.14 77.89,71.98 77.89,69.85 77.74,69.85 77.59,69.7 v77.59,65.55 v77.58,65.55 | IC1.41 67.81,59.76 69.39,61.34 69.39,63.82 68.91,64.29 68.91,65.09 69.23,65.41 69.39,65.41 v69.73,65.74
  Top 0.305: 77.59,79.76 77.74,79.91 77.74,80.06 77.89,80.21 v77.89,85.24 | v38.88,79.15 v38.88,85.24 | v18.15,65.58 18,65.43 16.78,65.43 v16.78,65.58 | v27.52,79.1 31.31,79.1 v31.41,78.99 | v23.94,72.75 23.94,65.58 21.05,65.58 20.89,65.43 20.89,64.36 19.52,64.36 19.37,64.52 v19.37,64.67 | 14.62,72.23 14.7,72.23 v14.95,71.98
  Bottom 0.152: v77.58,65.55 70.2,65.55 70,65.74 v69.73,65.74
  Bottom 0.305: v38.88,85.24 v77.89,85.24 | v38.88,79.15 38.73,79.3 31.87,79.3 31.71,79.15 31.56,79.15 v31.41,78.99 | v23.94,72.75 v27.6,72.75 v27.52,79.1 | v19.37,64.67 19.37,65.58 v18.15,65.58 | v16.78,65.58 16.63,65.73 15.87,65.73 15.71,65.89 15.71,70.46 15.1,70.46 14.95,70.61 v14.95,71.98
AD31  (via drill 0.2, 0.3)
  Top 0.152: v3.83,72.55 5.09,71.28 | 64.94,84.02 64.94,80.21 65.09,80.06 65.09,73.51 | IC1.42 67.74,60.26 68.75,61.28 | 68.75,61.28 | 68.75,61.28 68.91,61.44 68.91,63.66 67.96,64.61 67.96,64.93 69.07,66.04 69.07,70.17 70.1,71.2 v70.1,73.2 | v3.54,76.66 3.54,74.75 v3.52,74.73
  Top 0.254: 5.09,71.28 X1.J3-D22
  Top 0.305: v5.04,89.66 13.58,89.66 13.58,93.47 13.73,93.62 14.95,93.62 15.1,93.47 17.39,93.47 17.39,96.22 17.54,96.37 21.2,96.37 v21.2,96.52 | v64.94,93.93 64.94,85.7 64.78,85.55 64.78,84.18 64.94,84.02 | 65.09,73.51 v64.94,73.36 | v32.95,95.6 32.82,95.73 31.92,95.73 31.13,96.52 31.13,100.97 v31.26,101.09
  Bottom 0.152: 2.45,82.65 2.45,77.59 3.38,76.66 v3.54,76.66
  Bottom 0.305: v3.52,74.73 3.67,74.73 3.67,72.75 3.83,72.59 v3.83,72.55 | 2.45,82.65 2.3,82.8 2.3,89.2 2.15,89.36 2.15,90.4 2.24,90.49 4.78,90.49 4.94,90.33 4.94,89.77 v5.04,89.66 | v21.2,96.52 21.05,96.67 21.05,99.72 21.2,99.87 21.35,99.87 21.5,100.03 21.5,100.18 21.66,100.33 21.81,100.33 21.96,100.48 21.96,100.64 22.57,101.24 29.43,101.24 29.58,101.09 v31.26,101.09 | v32.95,95.6 32.63,93.93 v64.94,93.93 | v64.94,73.36 67.95,73.36 | v70.1,73.2 70,73.1 68.2,73.1 67.95,73.36 | 67.95,73.36
AREF  (via drill 0.3)
  Top 0.152: IC1.98 49.47,53.26 v49.86,53.66 | 60.18,96.84 60.18,95.41 59.39,94.62 59.39,80.7 59.66,80.43 59.66,75.92 | 56.21,71.44 56.21,70.01 56.53,69.69 56.53,68.62 v56.31,68.4
  Top 0.305: C6.2 61.61,102.08 59.55,100.01 59.55,97.47 60.18,96.84 | v56.85,63.98 56.21,63.98 55.74,63.5 v55.74,57.15 | v55.9,72.07 55.9,71.75 56.21,71.44 | v59.23,73.66 59.23,74.41 59.63,74.81 59.63,75.88 59.66,75.92
  Bottom 0.152: v56.85,63.98 56.05,64.77 | 56.05,67.63 56.31,67.89 v56.31,68.4
  Bottom 0.254: 56.05,72.39 57.32,73.66 v59.23,73.66 | 56.05,72.39 | 55.9,72.23 56.05,72.39 | 56.05,64.77 56.05,67.63
  Bottom 0.305: v49.86,53.66 49.86,56.52 50.5,57.15 v55.74,57.15 | v55.9,72.07 55.9,72.23
C/BE0#  (via drill 0.2, 0.3)
  Top 0.254: X1.J3-A4 11.14,35.25 18.91,35.25 19.07,35.41 v34,35.41
  Top 0.305: v60.98,66.19 60.21,66.19 IC1.51 | v60.21,58.05 v60.21,64.06 | v54.27,33.73 55.49,33.73 55.64,33.88 55.64,35.41 55.49,35.56 55.49,39.12 55.9,39.53 55.9,40.24 v56.85,41.2 | v60.34,41.27 60.68,41.27 60.9,41.49 60.9,51.2 60.52,51.58 60.52,53.16 v60.5,53.18
  Bottom 0.254: v34,35.41 40.17,35.41 41.13,34.45 41.58,34.45 41.62,34.49
  Bottom 0.305: v60.98,66.19 60.82,66.04 60.37,66.04 60.21,65.89 v60.21,64.06 | v54.27,33.73 54.12,33.88 46.04,33.88 45.89,33.73 45.89,33.58 44.82,33.58 44.67,33.73 44.67,34.49 41.62,34.49 | v56.85,41.2 60.26,41.2 v60.34,41.27 | v60.5,53.18 60.5,57.76 v60.21,58.05
C/BE1#  (via drill 0.2, 0.3)
  Top 0.152: 9.1,43.69 10.1,44.69 10.1,45.72 10.57,46.2 11.76,46.2 12.32,45.64 16.53,45.64 17.16,45.01 30.57,45.01 v30.73,45.17 | IC1.52 59.65,70.1 v59.6,70.16
  Top 0.254: X1.J3-B8 9.1,43.69
  Top 0.305: v49.7,73.34 48.58,73.36 39.7,73.36 39.24,73.82 38.59,73.82 38.27,73.5 34.62,73.5 34.15,73.03 v34.15,72.55
  Bottom 0.152: v30.73,45.17 30.73,47.38 30.81,47.47 30.81,54.77 31.61,55.56 32.08,56.04 | 32.08,56.04 | 32.08,56.04 32.24,56.2 | 32.24,60.48 33.67,61.91 33.67,64.14 33.99,64.45 33.99,72.39 v34.15,72.55 | 51.77,70.64 54.78,70.64 | v59.6,70.16 57.81,70.16 57.48,70.48 54.94,70.48 54.78,70.64 | 54.78,70.64
  Bottom 0.305: v49.7,73.34 51.37,71.68 51.37,71.04 51.77,70.64 | 32.24,56.2 32.24,60.48
C/BE2#  (via drill 0.3)
  Top 0.152: 5.09,55.25 6.05,56.2 | 6.13,56.2 6.13,57.86 6.44,58.18 9.78,58.18 10.02,58.42 | 10.1,58.5 10.1,59.93 10.33,60.17 11.6,60.17 11.92,59.85 12.3,59.85 12.66,59.49 13.02,59.49 13.13,59.37 v25.26,59.37 | 36.37,67.94 36.53,68.1 39.38,68.1 40.02,68.74 50.02,68.74 50.18,68.58 50.5,68.58 50.65,68.43 IC1.70
  Top 0.254: X1.J3-D14 5.09,55.25 | 6.05,56.2 6.13,56.2 | 10.02,58.42 | 10.02,58.42 10.1,58.5 | 13.13,59.37 15.73,59.37 | 29.86,62.71 v30.34,62.71 | v30.34,67.94 30.97,67.94
  Top 0.305: v25.1,62.71 29.86,62.71 | 30.97,67.94 36.37,67.94
  Bottom 0.152: v30.34,67.94 | v30.34,67.94 30.5,67.94 | v25.1,62.71 25.1,59.53 v25.26,59.37
  Bottom 0.254: v30.34,62.71 | v30.34,62.71 v30.34,67.94
C/BE3#  (via drill 0.2, 0.3)
  Top 0.152: X1.J3-B19 9.5,65.21 10.49,66.2 11.6,66.2 12.56,65.4 | IC1.28 68.36,53.26 68.59,53.02 69.23,53.02 69.71,53.5 v69.71,54.45 | v72.98,57.96 72.98,57.88 72.41,57.31 | 72.41,57.31
  Top 0.254: 18.46,64.82 16.47,64.82 15.9,65.4 12.56,65.4
  Top 0.305: v26.84,69.7 26.84,67.63 27.16,67.31 27.18,67.31 27.24,67.25 31.55,67.25 31.56,67.26 36.58,67.26 36.88,67.56 39.8,67.56 40.34,68.1 42.2,68.1 43.12,67.19 43.12,64.49 v41.92,63.3 | 72.41,57.31 v72.41,54.61 | 18.46,64.82 18.76,64.82 18.76,66.8 18.91,66.95 20.89,66.95 21.05,67.11 21.05,67.26 21.2,67.41 21.35,67.41 21.5,67.56 21.5,67.72 21.66,67.87 21.81,67.87 21.96,68.02 21.96,68.17 22.11,68.33 22.27,68.33 22.42,68.48 22.42,68.63 22.57,68.78 22.72,68.78 22.88,68.94 22.88,69.09 23.03,69.24 23.18,69.24 v23.18,69.55
  Bottom 0.152: v69.71,54.45 70.02,54.45 70.18,54.61 v72.41,54.61 | 71.07,60.55 71.22,60.55 71.61,60.17 | 71.61,60.17 | 71.61,60.17 72.98,58.8 v72.98,57.96
  Bottom 0.305: 71.07,60.55 56.42,60.55 55.79,59.92 46.95,59.92 46.8,60.55 46.8,61.16 46.65,61.32 46.5,61.32 46.34,61.47 46.34,61.62 46.19,61.77 46.04,61.77 45.89,61.92 45.89,62.08 45.73,62.23 45.58,62.23 45.43,62.38 45.43,62.53 45.28,62.69 42.54,62.69 42.38,62.84 42.08,62.84 41.92,62.99 v41.92,63.3 | v26.84,69.7 26.69,69.85 23.64,69.85 23.48,69.7 23.33,69.7 v23.18,69.55
CLK  (via drill 0.2)
  Top 0.152: IC1.34 63.49,56.26 63.79,55.96 70.19,55.96 v70.77,55.37
  Top 0.305: v73.17,55.37 73.17,33.12 QG1.3
  Bottom 0.305: v73.17,55.37 v70.77,55.37
CLK0  (via drill 0.3)
  Top 0.152: 9.22,79.21 10.18,80.17 11.76,80.17 12.24,79.69 15.41,79.69 15.57,79.85 | v46.85,65.88 46.85,65.72 47.16,65.41 | 26.69,73.82 26.69,71.28 27.16,70.8
  Top 0.254: X1.J3-B26 9.22,79.21 | 15.57,79.85 16.21,79.85 16.53,79.53 19.52,79.53 19.54,79.53
  Top 0.305: IC1.23 59.15,51.99 v58.59,52.55 58.12,53.02 57.48,53.66 52.88,53.66 50.97,55.56 50.97,62.86 49.07,64.77 47.8,64.77 47.16,65.41 | 27.16,70.8 34.15,70.8 v35.73,72.39 | v26.69,76.68 26.69,73.82 | v37.96,74.61 39.54,74.61 40.02,74.14 43.67,74.14 v44.15,74.61 | 19.52,79.53 19.52,79.45 19.68,79.3 19.68,79.15 19.83,78.99 21.2,78.99 21.2,77.47 21.5,77.17 23.33,77.17 23.33,76.71 v23.35,76.68
  Bottom 0.152: v44.15,74.61 44.15,65.88 44.31,65.72 44.78,65.72 44.94,65.88 v46.85,65.88
  Bottom 0.305: v23.35,76.68 v26.69,76.68 | v35.73,72.39 v37.96,74.61
CLK1  (via drill 0.3)
  Top 0.152: v25.73,67.94 26.05,68.26 26.05,75.41 25.73,75.72 v25.57,75.72
  Top 0.254: v12.87,78.11 16.21,78.11 16.53,78.42 18.91,78.42
  Top 0.305: v25.57,65.88 v41.45,65.88 | IC1.24 59.65,52.76 58.75,53.66 58.12,54.29 53.36,54.29 51.77,55.88 v51.77,64.45 | 18.91,78.42 18.91,78.54 20.74,78.54 20.74,77.17 20.89,77.01 20.89,76.86 21.05,76.71 22.57,76.71 22.57,75.95 22.72,75.79 23.33,75.79 v23.35,75.64
  Bottom 0.152: 5.26,79.21 6.29,78.18 12.79,78.18 v12.87,78.11 | v23.35,75.64 23.43,75.72 v25.57,75.72
  Bottom 0.254: 5.26,79.21 X1.J3-D26
  Bottom 0.305: v25.73,67.94 25.73,66.04 v25.57,65.88 | 51.45,64.14 47.16,64.14 46.69,64.61 43.99,64.61 42.72,65.88 v41.45,65.88 | 51.45,64.14 | 51.45,64.14 v51.77,64.45
CLK2  (via drill 0.2, 0.3)
  Top 0.152: IC1.25 60.15,48.86 v59.7,48.42
  Top 0.305: v63.11,49.89 65.24,47.75 v65.85,47.75 | v77.59,50.8 v77.59,47.75 | v81.24,50.95 81.24,52.48 81.4,52.63 81.4,53.24 82.01,53.85 v82.01,55.22 | v84.45,55.22 84.9,54.76 v84.9,51.87 | v97.86,52.32 97.86,56.9 v97.7,57.05 | v94.05,57.35 94.05,59.33 94.2,59.49 94.2,60.71 94.05,60.86 94.05,61.77 94.5,62.23 v94.5,66.19 | v86.73,68.17 v86.73,66.19 | v85.51,68.17 85.66,68.33 85.66,74.88 85.51,75.03 v85.51,82.19 | v75.15,82.19 75.3,82.35 75.3,86.31 v75.15,86.46 | v53.05,87.07 v53.05,85.85 | v35.52,87.38 35.37,87.22 35.37,84.48 v35.52,84.33 | v30.8,81.74 30.65,81.89 28.06,81.89 28.06,81.13 v27.6,80.67 | v23.79,80.67 23.79,79.76 23.48,79.45 20.89,79.45 v20.89,82.04 | v19.07,81.89 18.46,81.28 17.24,81.28 17.08,81.43 15.1,81.43 v15.1,81.59 | v55.18,85.85 55.18,83.71 v55.95,82.94 | v63.72,86.46 63.72,86.25 63.52,86.04 63.52,82.82 v63.56,82.78
  Bottom 0.152: v63.11,49.89 61.64,48.42 v59.7,48.42
  Bottom 0.305: v65.85,47.75 71.49,47.75 71.64,47.6 77.43,47.6 v77.59,47.75 | v77.59,50.8 77.74,50.95 v81.24,50.95 | v82.01,55.22 82.16,55.37 83.83,55.37 83.99,55.22 v84.45,55.22 | v84.9,51.87 85.05,52.02 97.55,52.02 v97.86,52.32 | v97.7,57.05 97.4,57.35 v94.05,57.35 | v86.73,66.19 v94.5,66.19 | v85.51,68.17 v86.73,68.17 | v85.51,82.19 85.36,82.35 75.3,82.35 v75.15,82.19 | v53.05,85.85 v55.18,85.85 | v53.05,87.07 52.9,86.92 39.79,86.92 39.64,87.07 37.66,87.07 37.51,87.22 36.59,87.22 36.44,87.38 v35.52,87.38 | v35.52,84.33 34.3,83.11 31.87,83.11 30.8,82.04 v30.8,81.74 | v23.79,80.67 v27.6,80.67 | v20.89,82.04 20.74,81.89 v19.07,81.89 | v15.1,81.59 14.95,81.74 12.82,81.74 12.36,81.28 11.14,81.28 X1.J3-A27 | v55.95,82.94 63.4,82.94 v63.56,82.78 | v63.72,86.46 v75.15,86.46
CLK3  (via drill 0.2, 0.3)
  Top 0.152: 19.54,80.33 19.56,80.33 | v69.66,51.56 69.57,51.65 62.92,51.65 62.61,51.96 62.45,51.96 IC1.26 | v12.71,80.57 15.81,80.57 15.89,80.49
  Top 0.254: 15.89,80.49 16.53,80.49 16.68,80.33 19.52,80.33 19.54,80.33
  Top 0.305: v77.13,51.56 76.98,51.71 76.98,54.61 v77.13,54.76 | v79.72,54.76 79.57,54.92 79.57,59.49 79.72,59.64 79.72,69.55 79.87,69.7 80.03,69.7 80.03,70.61 79.87,70.76 79.72,70.76 79.72,72.44 79.42,72.75 79.42,79.3 79.72,79.6 79.72,84.48 79.87,84.63 79.87,85.7 80.03,85.85 v80.03,89.66 | v25.47,85.09 25.47,80.21 v25.31,80.06 | v33.24,89.66 33.24,84.66 33.19,84.61 28.08,84.61 v27.6,85.09 | v21.96,80.21 23.18,80.21 v23.18,80.06 | 19.52,80.33 v19.52,80.21
  Bottom 0.152: 7.15,81.21 8.19,80.17 12.32,80.17 v12.71,80.57
  Bottom 0.254: X1.J3-C27 7.15,81.21 | v69.66,51.56 69.95,51.28 76.69,51.28 76.98,51.56 v77.13,51.56
  Bottom 0.305: v79.72,54.76 v77.13,54.76 | v80.03,89.66 79.87,89.81 73.62,89.81 72.86,89.05 61.89,89.05 61.74,89.2 61.74,89.81 33.39,89.81 v33.24,89.66 | v25.47,85.09 v27.6,85.09 | v23.18,80.06 v25.31,80.06 | v19.52,80.21 v21.96,80.21
DEVSEL#  (via drill 0.2, 0.3)
  Top 0.152: v28.91,92.08 28.91,93.5 v29.07,93.66 | v75.61,75.18 75.45,75.03 75.45,71.22 | v11.92,54.21 14.7,54.21 17.32,51.59 | 17.32,51.59 | 17.32,51.59 18.43,50.48 18.83,50.48 20.02,49.29 23.35,49.29 23.58,49.52 v23.86,49.52 | v57.32,71.07 57.64,70.75 57.64,68.26 57.32,67.94 57.32,67.79 57.15,67.61 IC1.57
  Top 0.305: v75.61,71.07 75.45,71.22 | v54.12,73.2 54.27,73.36 54.27,88.14 54.42,88.29 54.42,92.91 53.83,93.5 30.5,93.5 v30.34,93.34
  Bottom 0.152: 5.09,51.28 6.05,52.23 6.05,53.9 6.36,54.21 v11.92,54.21 | v29.07,93.66 29.7,93.66 v30.34,93.34 | v75.61,75.18 82.16,75.18 | 59.55,70.96 69.4,70.96 | v28.91,92.08 28.91,91.6 28.75,91.44 28.75,72.23 28.11,71.6 28.11,68.9 27.96,68.74 27.96,58.42 25.97,56.44 25.97,51.81
  Bottom 0.254: X1.J3-D12 5.09,51.28 | v57.32,71.07 58.33,71.07 58.59,70.8 59.39,70.8 59.55,70.96 | 69.4,70.96 69.51,71.07
  Bottom 0.305: v75.61,71.07 75.45,71.22 69.66,71.22 69.51,71.07 | 82.16,75.18 R1.7 | 54.94,71.44 54.94,72.23 54.12,73.06 v54.12,73.2 | 54.94,71.44 | 25.97,51.81 25.97,51.63 v23.86,49.52 | 54.94,71.44 55.26,71.12 | 55.26,71.12 | 55.26,71.12 55.31,71.07 v57.32,71.07
FRAME#  (via drill 0.2, 0.3)
  Top 0.152: X1.J3-A13 12.27,53.21 12.56,53.5 14.7,53.5 16.88,51.32 | IC1.53 59.15,69.36 58.99,69.51 58.99,70.56 59.39,70.96 | 16.88,51.32 17.08,51.12 | 76.98,70.16 76.98,62.69 | v29.7,95.41 29.7,91.59 v29.85,91.44 | v24.8,48.97 24.65,48.82 19.62,48.82 18.43,50.01 18.19,50.01 16.88,51.32 | v60.94,70.31 61.29,70.66 61.29,72.39 60.98,72.71 60.88,72.71 | 59.39,70.96 | 59.39,70.96 59.86,71.44 59.86,72.23 60.5,72.87 60.72,72.87 60.88,72.71 | v60.88,87.51 60.88,72.71 | 16.88,51.32
  Top 0.305: 76.98,62.69 v77.13,62.53 | v77.13,70.31 76.98,70.16 | v55.64,87.53 55.64,96.14 55.26,96.52 | v32.08,96.68 32.24,96.84 42.24,96.84 42.4,97 54.78,97 55.26,96.52 | 55.26,96.52
  Bottom 0.152: v77.13,62.53 82.16,62.53 | v29.85,91.44 29.38,91.44 29.23,91.28 29.23,72.07 28.59,71.44 28.59,68.74 28.43,68.58 28.43,58.1 27.96,57.63 | 27.96,57.63 | 27.8,57.47 27.96,57.63 | 27.8,57.47 | 26.53,56.2 27.8,57.47 | 26.53,51.12 24.8,49.4 v24.8,48.97 | 69.66,70.46 61.1,70.46 v60.94,70.31
  Bottom 0.305: v29.7,95.41 30.81,95.41 31.61,96.2 31.77,96.2 v32.08,96.68 | v77.13,70.31 75.15,70.31 75,70.46 75,70.61 69.81,70.61 69.66,70.46 | 82.16,62.53 R1.2 | v55.64,87.53 v60.88,87.51 | 26.53,51.12 26.53,56.2
GND  (via drill 0.2, 0.3)  (1 unrouted)
  Top 0.152: X1.J3-D11 X1.J3-C12 7.09,51.61 8.03,52.55 8.11,52.63 | 8.11,52.63 8.11,54.05 8.19,54.13 8.27,54.21 10.1,54.21 X1.J3-A14 | X1.J3-D20 3.98,68.32 3.98,70.01 | 4.14,70.17 6.13,70.17 7.09,71.14 | 11.13,75.25 v17.48,75.25 | X1.J3-B23 X1.J3-C22 6.13,72.18 6.13,75.8 5.09,76.84 | 5.09,77.31 3.67,78.74 3.67,79.78 X1.J3-D27 X1.J3-C26 | 11.92,46.99 12.4,46.51 v14.94,46.51 | 8.11,52.63 8.19,52.63 8.59,53.02 8.91,53.02 X1.J3-B13 | v58.75,75.25 58.59,75.41 | X1.J3-A28 17.29,83.21 v17.48,83.03 | 52.56,52.94 52.56,53.02
  Top 0.254: X1.J3-A20 11.63,66.67 14.46,66.67 14.78,66.36 v17.48,66.36 | 4.14,70.17 3.98,70.01 | X1.J3-C22 7.09,71.14 | X1.J3-A24 11.13,75.25 | 5.09,76.84 X1.J3-D25 5.09,77.31 | X1.J3-D27 5.09,81.28 | v53.12,52.39 53.15,52.36 IC1.11 53.15,48.05 v52.88,47.78 | 8.03,52.55 | 8.19,54.13
  Top 0.305: X1.J3-C4 X1.J3-D5 5.04,37.39 5.04,39.06 X1.J3-D6 X1.J3-C7 | C3.1 54.65,71.73 IC1.62 54.65,63.84 v54.31,63.5 | IC3.7 67.98,18.34 67.98,15.75 69.36,14.38 69.36,12.7 C18.- | v68.59,27.03 68.59,25.81 IC3.21 | IC3.18 70.58,25.81 v70.58,27.03 70.58,29.31 71.95,29.31 72.1,29.16 73.02,29.16 QG1.2 | C2.2 42.54,103.07 42.54,107.64 42.38,107.8 40.71,107.8 40.71,109.47 J3.5 40.71,109.63 40.71,112.06 J3.6 | v81.55,103.07 81.55,109.47 J8.9 | J2.6 J2.5 22.88,104.75 22.72,104.6 22.11,104.6 22.11,102.92 C4.2 | v90.24,71.83 90.24,68.94 LED1.C | v83.99,66.95 83.99,56.13 83.83,55.98 83.53,55.98 83.53,54.3 C33.2 | C34.2 77.89,20.32 77.89,14.07 77.74,13.92 75.61,13.92 75.61,12.24 C14.1 | C18.- 69.36,12.55 | C35.2 82.01,31.45 82.01,29.77 81.85,29.62 80.64,29.62 80.64,25.81 C16.1 80.64,25.65 80.64,23.22 80.48,23.06 80.48,20.47 v80.64,20.32 | 93.44,29.62 89.78,29.62 89.63,29.46 89.63,25.96 C15.2 | 93.44,29.62 93.44,31.45 C31.2 | 95.88,26.42 98.31,26.42 | 98.31,26.42 101.97,26.42 102.12,26.26 102.12,23.52 101.97,23.37 101.82,23.37 101.67,23.22 101.67,23.06 101.51,22.91 101.36,22.91 101.21,22.76 101.21,22.15 101.06,22 101.06,21.84 100.29,21.84 X2.GND | 95.88,26.42 95.88,25.81 C19.2 | 98.31,36.47 100.14,36.47 100.29,36.63 100.29,40.13 J7.5 | 98.31,26.42 98.31,36.47 | 93.44,29.62 94.35,29.62 94.35,27.33 94.5,27.18 94.66,27.18 94.81,27.03 95.88,27.03 95.88,26.42 | 98.31,36.47 98.16,36.63 98.16,51.71 96.03,51.71 95.88,51.87 95.88,53.54 J5.1 | v53.36,40.16 53.36,38.1 C7.2 | v63.36,41.43 63.36,35.56 64.15,34.77 64.47,34.77 64.78,34.45 64.78,27.46 65.22,27.03 v66,27.03 66,25.81 IC3.25 66,25.65 v66,23.37
  Top 0.305: v49.23,61.75 46.85,61.75 46.8,61.77 46.19,61.77 IC1.81 | v54.31,61.75 54.31,58.42 v54.62,58.1 | v56.85,56.52 57.16,56.2 59.7,56.2 60.64,55.26 IC1.32 | v44.67,16.66 44.67,7.67 X3.5 | v23.48,18.03 23.48,16.81 C27.- 23.48,16.51 v23.48,10.11 | v31.87,18.03 31.87,16.81 C26.- | v40.4,18.03 40.4,16.81 C25.- | v87.64,32.97 C10.2 | v69.51,7.67 69.36,7.82 69.36,12.39 C18.- | v46.5,23.22 46.5,16.97 C24.+ | 58.59,75.41 58.59,76.04 59.13,76.46 59.13,80.38 58.84,80.67 58.84,96.06 C5.2 58.84,96.22 58.84,100.94 58.99,101.09 59.15,101.09 59.15,102.77 C6.1 59.3,103.1 59.3,104.6 59.86,105.16 59.86,110.81 58.61,112.06 58.54,112.06 | IC1.99 50.08,52.76 50.66,53.34 52.24,53.34 52.56,53.02 | v53.12,52.39 52.56,52.94 | X1.J3-B9 9.1,45.59 10.49,46.99 10.88,46.99 X1.J3-A10 11.7,47.21 11.92,46.99 | 58.54,112.06 58.38,112.06 | 58.54,112.06 J1.6
  Bottom 0.152: 10.1,36.12 10.1,34.21 X1.J3-B3 X1.J3-C4 | 10.18,36.29 X1.J3-A5 | 9.11,33.21 10.1,32.23 10.1,30.21 X1.J3-A1 | X1.J3-C7 8.11,42.23 8.11,44.23 X1.J3-B9 | 5.09,48.74 4.14,47.78 4.14,46.67 3.51,46.04 3.51,43.97 3.98,43.5 3.98,40.32 X1.J3-D6 | X1.J3-D15 X1.J3-C16 8.12,58.18 9.62,58.18 10.1,57.71 10.1,56.59 11.1,55.59 X1.J3-A14 | 7.09,59.63 8.11,60.64 8.11,62.23 X1.J3-B18 | X1.J3-B23 X1.J3-A24 | C29.2 22.08,92.87 21.29,92.08 C28.2 | v17.48,66.36 17.48,64.93 17.64,64.77 17.64,54.77 16.05,53.18 16.05,47.47 15.1,46.51 v14.94,46.51 | v54.31,61.75 v54.31,63.5 | v58.75,75.25 58.02,75.25 57.93,75.34 | X1.J3-D27 6.09,82.2 6.09,86.32 5.2,87.21 X1.J3-D30 | v17.48,75.25 v17.48,83.03
  Bottom 0.254: 10.1,36.12 10.18,36.2 10.18,36.29 | X1.J3-B3 9.11,33.21 | X1.J3-C7 | 5.09,48.74 X1.J3-D11 | X1.J3-C16 7.09,59.63 | v17.48,75.25 v17.48,66.36
  Bottom 0.305: v66,27.03 v68.59,27.03 v70.58,27.03 70.73,27.18 73.02,27.18 73.17,27.03 79.87,27.03 80.03,26.87 80.03,25.65 80.64,25.65 C16.1 | C9.2 65.7,96.22 64.02,96.22 63.87,96.06 63.87,95.15 60.98,95.15 60.82,95.3 60.21,95.3 60.06,95.45 60.06,96.22 58.99,96.22 C5.2 | v81.55,103.07 68.29,103.07 C17.2 68.14,103.07 67.68,103.07 67.53,103.23 67.53,103.84 66.77,103.84 66.61,103.99 66.31,103.99 66.16,104.14 65.39,104.14 65.24,103.99 60.21,103.99 60.06,103.84 60.06,102.92 59.15,102.92 C6.1 59.02,102.92 57.32,102.92 57.16,102.77 55.49,102.77 C32.2 55.34,102.77 54.27,102.77 54.27,101.4 54.12,101.24 44.21,101.24 | 44.21,101.24 44.21,102.92 44.06,103.07 42.69,103.07 C2.2 | 44.21,101.24 44.21,100.33 39.79,100.33 39.64,100.48 34.3,100.48 34.15,100.64 34.15,101.24 32.32,101.24 32.17,101.4 32.17,102.62 30.95,102.62 30.8,102.77 30.65,102.77 30.65,102.92 30.5,103.07 29.89,103.07 C1.2 29.73,103.07 28.82,103.07 28.67,102.92 28.67,102.31 28.36,102.31 28.21,102.16 27.9,102.16 27.75,102.01 22.95,102.01 C4.2 20.81,101.6 20.34,101.6 19.86,101.12 19.86,96.68 20.02,96.52 20.02,96.04 | C8.2 48.02,38.46 49.39,38.46 49.55,38.61 49.55,39.37 52.56,39.37 v53.36,40.16 | 91.76,71.83 94.05,71.83 94.2,71.98 94.2,73.66 J4.1 97.7,73.66 97.7,73.36 97.86,73.2 100.29,73.2 J6.5 | 91.76,71.83 v90.24,71.83 | 82.46,52.48 82.46,54.3 83.38,54.3 C33.2 | 82.46,52.48 82.46,49.28 82.31,49.12 81.55,49.12 IC2.15 | 82.46,52.48 90.84,52.48 90.84,53.54 91,53.7 95.88,53.7 J5.1 | 91.76,71.83 91.76,66.65 89.93,66.65 89.78,66.8 89.78,66.95 v83.99,66.95 | C18.- 69.51,12.7 71.19,12.7 71.19,12.39 71.34,12.24 75.45,12.24 C14.1 75.61,12.24 76.67,12.24 76.67,14.22 76.83,14.38 82.31,14.38 C30.2
  Bottom 0.305: C35.2 82.01,31.6 82.62,31.6 82.77,31.75 82.77,32.82 83.22,32.82 83.38,32.97 v87.64,32.97 91.45,32.97 91.61,32.82 91.61,31.6 93.28,31.6 C31.2 | v80.64,20.32 C34.2 | 57.93,75.34 57.77,75.49 53.66,75.49 53.51,75.34 53.51,73.66 53.36,73.51 52.9,73.51 C3.1 | v52.88,47.78 52.88,47.31 53.2,46.99 53.2,40.32 v53.36,40.16 | v63.36,41.43 63.2,41.43 62.72,40.96 | 62.72,40.96 | 62.72,40.96 62.24,40.48 61.13,40.48 60.98,40.32 53.51,40.32 v53.36,40.16 | v54.31,61.75 v49.23,61.75 | v54.62,58.1 56.53,58.1 56.85,57.78 v56.85,56.52 55.1,54.77 53.36,54.77 53.2,54.61 53.2,52.47 v53.12,52.39 | X1.J3-D30 5.89,88 5.89,88.27 6.05,88.42 6.05,89.06 6.84,89.85 7.32,89.85 7.63,90.17 7.63,91.12 12.56,96.04 | 12.56,96.04 | C25.- 40.4,16.66 v44.67,16.66 44.82,16.81 46.5,16.81 C24.+ | JP13.3 12.05,10.11 16.78,10.11 JP12.3 16.93,10.11 v23.48,10.11 | v23.48,18.03 v31.87,18.03 v40.4,18.03 | v69.51,7.67 67.53,7.67 S1.1 | v46.5,23.22 46.65,23.37 v66,23.37 | C29.2 20.65,94.46 20.65,95.41 20.02,96.04 | 20.02,96.04 12.56,96.04
  pour Bottom (isolate 0.305): 0.01,116.2 108.6,115.57 109.23,-0.64 0.65,0
GNT0#  (via drill 0.3)
  Top 0.152: v28.11,99.7 v16.53,99.7 | 41.53,50.09 28.21,50.09 27.97,50.32 23.35,50.32 23.02,49.99 v22.91,49.99
  Top 0.254: IC1.97 45.2,53.76 41.53,50.09
  Top 0.305: v6.52,91.44 9.22,91.44 10.33,92.55 10.33,95.41 v11.45,96.52
  Bottom 0.152: 28.19,93.5 28.19,99.57 28.19,99.62 | 28.19,93.5 | 28.19,93.5 28.19,72.31 27.64,71.75 27.64,69.06 27.4,68.82 27.4,58.66 26.84,58.1 | 26.84,58.1 | 26.84,58.1 25.41,56.67 25.41,52.39 | v22.91,49.99 23.02,49.99 | X1.J3-D24 4.18,75.21 3.83,75.56 2.63,75.56 1.78,76.42
  Bottom 0.305: 23.02,49.99 25.41,52.39 | v28.11,99.7 28.21,99.57 28.19,99.57 | 1.78,76.42 1.78,82.21 1.44,82.55 1.44,90.96 1.76,91.28 6.36,91.28 v6.52,91.44 | v11.45,96.52 11.92,96.52 12.18,96.78 14.62,96.78 16.53,98.68 v16.53,99.7
GNT1#  (via drill 0.2, 0.3)
  Top 0.152: v20.02,52.39 21.45,50.96 21.53,50.88 41.69,50.88 | X1.J3-A25 11.55,77.21 12.24,76.52 13.99,76.52
  Top 0.254: 13.99,76.52 16.37,76.52 16.84,76.99 18.11,76.99 18.59,76.52 | 41.69,50.88 45.07,54.26 IC1.96
  Top 0.305: v19.83,74.73 19.83,75.95 19.22,75.95 19.07,76.1 19.07,76.25 18.91,76.4 18.61,76.4 18.59,76.52
  Bottom 0.152: 20.02,71.91 v20.02,52.39
  Bottom 0.305: 20.02,71.91 20.02,74.61 19.98,74.73 v19.83,74.73
GNT2#  (via drill 0.2, 0.3)
  Top 0.152: 7.3,77.21 8.27,78.18 11.68,78.18 12.71,77.15 14.14,77.15 | 41.61,51.44 22.24,51.44 21.11,52.56 v21.11,52.72 | 44.94,54.77 44.95,54.76
  Top 0.254: 7.3,77.21 X1.J3-C25 | 14.14,77.15 16.05,77.15 16.53,77.63 18.43,77.63 18.9,77.16 18.91,77.15 | 41.61,51.44 44.94,54.77 | 44.95,54.76 IC1.95
  Top 0.305: v20.74,73.2 20.59,73.2 20.44,73.36 20.44,75.03 20.28,75.18 20.28,76.25 20.13,76.4 20.13,77.01 19.98,77.17 18.91,77.17 18.9,77.16
  Bottom 0.152: 20.81,73.18 20.79,73.16 20.65,73.03 20.65,53.17 v21.11,52.72
  Bottom 0.305: 20.79,73.16 v20.74,73.2
GNT3#  (via drill 0.3)
  Top 0.254: v14.78,92.55 14.94,92.55 15.57,91.92 15.57,91.76 18.11,89.22 | v22.32,53.97 22.32,52.78 23.03,52.07 | 23.03,52.07 | 23.03,52.07 23.11,51.99 | IC1.94 44.8,55.26 41.53,51.99
  Top 0.305: v23.83,89.22 18.11,89.22 | 23.11,51.99 41.53,51.99
  Bottom 0.152: v22.32,53.97 22.56,87.15
  Bottom 0.254: 8.52,90.9 10.65,93.03 14.3,93.03 v14.78,92.55
  Bottom 0.305: v23.83,89.22 23.83,88.74 23.35,88.27 23.03,88.27 22.56,87.79 22.56,87.15 | X1.J3-C30 7.09,87.57 7.95,88.42 7.95,89.38 8.59,90.01 8.59,90.84 8.52,90.9
IDSEL0  (via drill 0.2)
  Top 0.152: 23.95,52.63 41.53,52.63
  Top 0.254: X1.J3-A18 11.66,63.21 12.08,62.79 12.64,62.79 12.87,63.02 | 17.48,62.39 15.35,62.39 14.71,63.02 12.87,63.02 | IC1.93 44.66,55.76 41.53,52.63 | 12.87,63.02 | 19.52,54.76 22.7,54.76 22.72,54.77 | 22.72,54.77 | 22.72,54.77 23.19,54.29 23.19,53.66 22.95,53.42 22.95,53.1 23.35,52.7 | 23.35,52.7 | 23.35,52.7 23.43,52.63 23.95,52.63
  Top 0.305: v18.46,62.41 18.46,62.38 17.54,62.38 17.48,62.39 | v19.37,54.76 19.52,54.76
  Bottom 0.305: v18.46,62.41 18.46,54.76 v19.37,54.76
IDSEL1  (via drill 0.2)
  Top 0.152: X1.J3-C18 8.1,64.21 15.33,64.21 | 15.73,63.82 | 15.73,63.82 15.81,63.74
  Top 0.254: 15.33,64.21 15.73,63.82 | 15.81,63.74 18.27,63.74 18.99,63.02 | 41.61,53.34 44.53,56.26 IC1.92
  Top 0.305: 18.99,63.02 21.01,63.02 21.5,62.53 v21.5,62.49 | v23.94,53.39 23.99,53.34 41.61,53.34
  Bottom 0.254: 21.96,53.09 23.64,53.09
  Bottom 0.305: v21.5,62.49 21.5,53.54 21.96,53.09 | 23.64,53.09 v23.94,53.39
IDSEL2  (via drill 0.2, 0.3)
